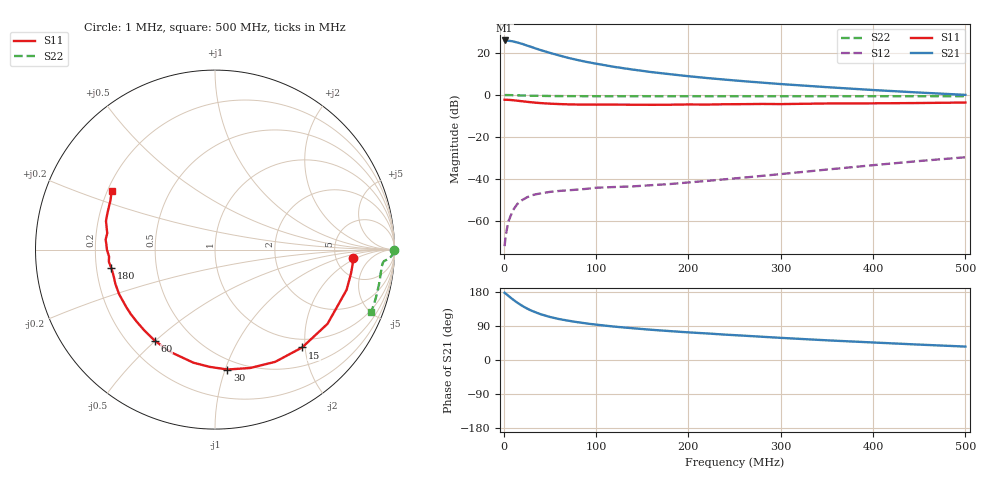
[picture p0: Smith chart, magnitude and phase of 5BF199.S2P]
! BF199, SILICON NPN RF TRANSISTOR IN TO92 PACKAGE
! distance from case: 2.5mm
! VCE=10V IC=10mA
# GHZ S MA R 50
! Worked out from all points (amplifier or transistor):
!   31 points, 1 MHz to 500 MHz, reference 50 ohm
!   highest |S21| = 26.0 dB at 1 MHz (marker M1)
!   |S21| within 3 dB of that: start of sweep to 29.31 MHz
!   unconditionally stable (mu >= 1): 111.2 MHz to 331 MHz
!   at 15 MHz: K = 0.20, MSG = 38.4 dB, |S12| = -51.8 dB
!   at 90 MHz: K = 0.88, MSG = 30.2 dB, |S12| = -44.7 dB
!   at 500 MHz: K = 0.50, MSG = 14.9 dB, |S12| = -29.7 dB
!   S11 on the Smith chart (normalised r, x): 1 MHz: 7.41, -1.63; 15 MHz: 0.83, -1.94; 30 MHz: 0.42, -1.02; 60 MHz: 0.31, -0.50; 180 MHz: 0.26, -0.08; 500 MHz: 0.22, +0.25
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0.001  0.772 -3.3  19.93 177.5  0.00025 81.6  0.997 -0.1
0.003  0.7691 -10.2  19.84 173.5  0.000553 85.5  0.9966 -0.5
0.005  0.7667 -17.0  19.65 169.5  0.00096 80.0  0.9952 -0.8
0.01  0.7511 -33.4  18.94 159.7  0.001793 74.5  0.9901 -1.6
0.015  0.7301 -48.3  17.75 150.8  0.002566 68.7  0.9825 -2.2
0.02  0.7096 -61.8  16.53 143.0  0.003131 65.0  0.9755 -2.7
0.025  0.6881 -73.5  15.14 136.1  0.003627 58.9  0.9683 -3.0
0.03  0.6717 -84.0  13.95 130.2  0.004054 56.0  0.963 -3.2
0.035  0.654 -92.6  12.77 125.5  0.004316 52.9  0.9576 -3.4
0.04  0.6415 -100.8  11.76 120.8  0.004514 51.7  0.9528 -3.6
0.05  0.622 -113.6  10.09 113.6  0.00491 50.2  0.9462 -3.8
0.06  0.6083 -123.5  8.767 108.0  0.005174 49.9  0.9424 -4.0
0.07  0.5982 -131.2  7.66 103.7  0.005362 50.7  0.9399 -4.3
0.09  0.5911 -142.4  6.125 96.3  0.005817 54.8  0.9366 -4.9
0.12  0.5892 -155.1  4.67 88.1  0.006423 58.9  0.9333 -5.8
0.16  0.5837 -165.8  3.516 79.7  0.007102 69.9  0.9333 -7.2
0.18  0.5867 -170.0  3.134 76.2  0.007562 75.2  0.9324 -8.0
0.22  0.5914 -176.2  2.54 70.1  0.008959 85.8  0.933 -9.6
0.26  0.6058 177.3  2.131 64.2  0.01075 95.3  0.9337 -11.3
0.35  0.6278 165.3  1.537 51.9  0.01672 109.7  0.9348 -15.1
0.45  0.6439 154.8  1.144 40.6  0.02671 117.4  0.9363 -19.6
0.5  0.6616 150.3  1.007 35.4  0.03288 119.2  0.9366 -21.9
